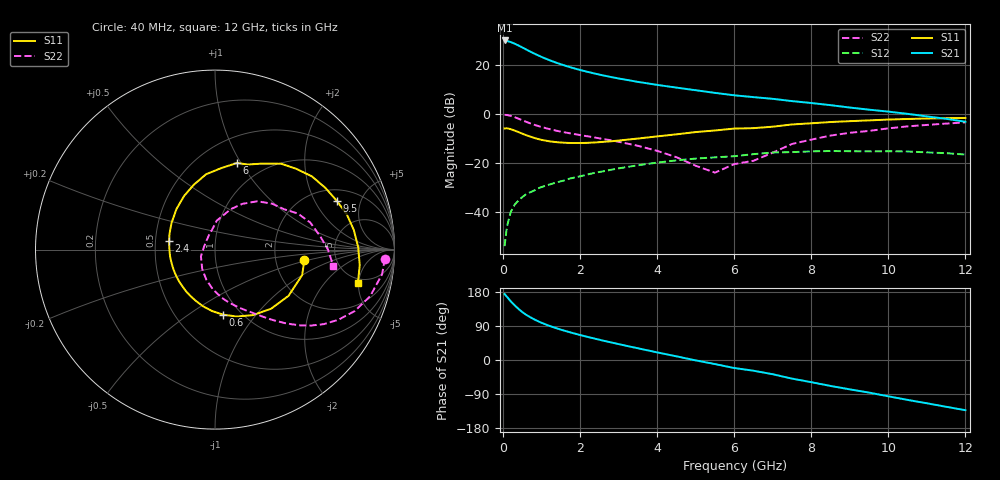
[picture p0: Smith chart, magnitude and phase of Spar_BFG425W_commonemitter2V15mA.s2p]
! Filename: 215bfg425.001
! BFG425W Field C1
! V1=8.558E-001V,V2=2.000E+000V, I1=2.081E-004A, I2=1.497E-002A
# GHz  S  MA  R 50
!  S11  S21  S12  S22
!Freq(GHz)  Mag  Ang  Mag  Ang  Mag  Ang  Mag  Ang
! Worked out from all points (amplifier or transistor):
!   44 points, 40 MHz to 12 GHz, reference 50 ohm
!   highest |S21| = 29.9 dB at 40 MHz (marker M1)
!   |S21| within 3 dB of that: start of sweep to 517.7 MHz
!   unconditionally stable (mu >= 1): 1.509 GHz to end of sweep
!   at 700 MHz: K = 0.67, MSG = 28.7 dB, |S12| = -32.0 dB
!   at 2.4 GHz: K = 1.14, MAG = 17.9 dB, |S12| = -24.0 dB
!   at 12 GHz: K = 1.36, MAG = 3.1 dB, |S12| = -16.7 dB
!   lowest NFmin = 1.60 dB at 900 GHz
!   S11 on the Smith chart (normalised r, x): 40 MHz: 2.93, -0.44; 600 MHz: 0.83, -0.69; 2.4 GHz: 0.59, +0.06; 6 GHz: 0.75, +0.96; 9.5 GHz: 2.63, +3.07; 12 GHz: 4.30, -4.89
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0.04  0.501 -6.5  31.09 174.1  0.002 70.6  0.948 -3.1
0.1  0.506 -16.3  30.32 166.9  0.005 84.3  0.941 -8.4
0.2  0.484 -32.1  28.8 154.8  0.01 76.4  0.903 -16.7
0.3  0.454 -46.5  26.77 144.4  0.014 71.1  0.85 -23.8
0.4  0.422 -59.8  24.55 134.9  0.017 66.2  0.791 -29.6
0.5  0.392 -72.1  22.39 126.4  0.02 63.3  0.735 -34.4
0.6  0.365 -82.9  20.35 119.3  0.023 61.0  0.683 -38.3
0.7  0.343 -92.6  18.55 113.2  0.025 59.0  0.638 -41.5
0.9  0.306 -109.9  15.58 102.7  0.03 56.6  0.565 -46.5
1  0.293 -117.6  14.36 98.2  0.032 55.8  0.535 -48.5
1.2  0.274 -131.2  12.37 90.2  0.036 54.1  0.487 -52.2
1.6  0.256 -154.6  9.594 77.1  0.044 51.4  0.417 -58.5
2.2  0.255 177.8  7.103 60.8  0.058 46.3  0.346 -68.1
2.4  0.26 169.6  6.527 55.9  0.063 44.3  0.325 -71.5
3.5  0.312 133.5  4.456 30.9  0.089 30.9  0.222 -93.1
4.5  0.38 108.2  3.401 9.7  0.112 16.5  0.13 -123.2
6  0.498 75.8  2.373 -21.2  0.136 -7.8  0.094 108.8
6.5  0.508 69.0  2.178 -28.3  0.15 -11.1  0.11 99.0
8.5  0.677 37.0  1.494 -68.5  0.174 -47.8  0.358 48.8
9.5  0.731 21.8  1.209 -86.0  0.171 -64.3  0.446 30.3
10.5  0.781 8.1  0.994 -105.3  0.17 -82.7  0.552 15.8
12  0.818 -13.3  0.686 -132.5  0.147 -112.2  0.666 -8.0
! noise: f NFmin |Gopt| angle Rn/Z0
900  1.6  0.11  -162.4  0.18
2000  1.9  0.13  -162.1  0.2
